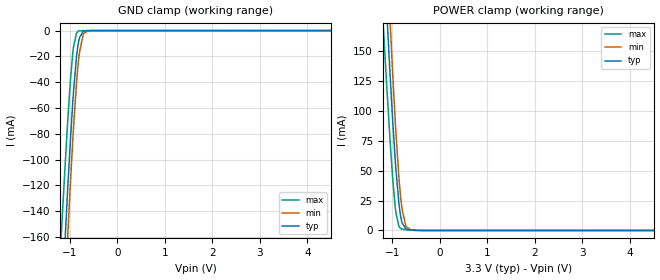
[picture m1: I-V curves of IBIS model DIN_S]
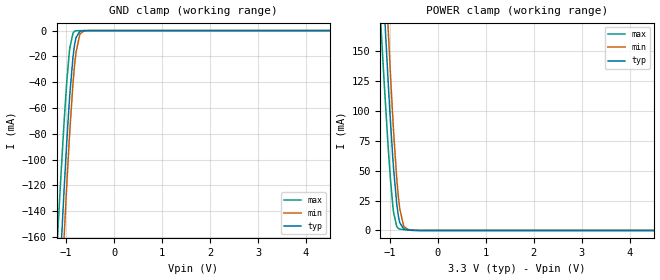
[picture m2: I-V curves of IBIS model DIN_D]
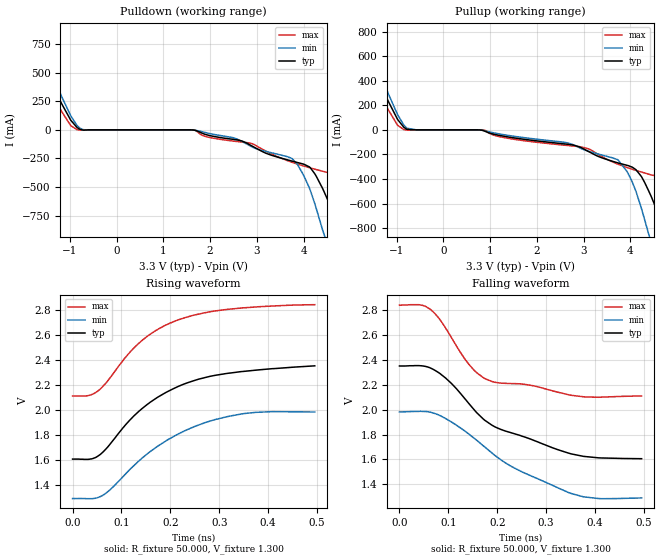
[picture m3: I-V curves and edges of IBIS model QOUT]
|Texas Instruments Incorporated
|3.3V  ECL 1:2 Fanout Buffer
|Valid for clock frequencies upto 2.4 - 2.9GHz
|*_S components are valid for parts used with D and DB in Single-Ended mode
|*_D components are valid for parts used with D and DB in Differential mode
| Marketing part#   Voltage Range   Package-type   #pins
|SN65LVEL11D   3.0V-3.8V   SOIC   8-pin
|SN65LVEL11DGK   3.0V-3.8V   MSOP(SOIC-TSSOP)   8-pin
[IBIS Ver]   4.0
[File name]   sn65lvel11.ibs
[File Rev]   1.1
[Date]   01/28/2009
[Source]   Texas Instruments Incorporated.
   Analog-eLab, HPA
   12500 TI Blvd
   Dallas, TX -75243
   For Support e-mail: elab_ibis@list.ti.com
[Notes]   Revision History:
   1.0: 01/27/2009
   - Model based on Simulations in TISPICE
   - Model not matched to silicon measurements
   1.1: 01/28/2009
   - Model updated with separate components and input_ECL models
   with *_S and *_D extensions. *_S valid for part configuration with
   D and DB as single-ended. *_D valid for part configuration with
   D and DB pair as differential
   - Updated ccomp, [pin] and [package] parasitics to be valid
   for speeds upto 2.9GHz
[Disclaimer]
 This product is designed as an aid for customers of Texas Instruments.
 No warranties, either expressed or implied, with respect to this third
 party software (if any) or with respect to its fitness for any
 particular purpose is claimed by Texas Instruments or the author. The
 software (if any) is provided solely on an "as is" basis. The entire
 risk as to its quality and performance is with the customer
[Copyright] (C) Copyright 2009 Texas Instruments Incorporated.
   All rights reserved.
|   SN65LVEL11D_S for D/DB configured as Single-ended
[Component]   SN65LVEL11D_S
[Manufacturer]  Texas Instruments Incorporated
[Package]   |8-pin SOIC
|   typ   min   max
R_pkg   0.317   0.222   0.412
L_pkg   2.169nH   1.866nH   2.472nH
C_pkg   0.429pF   0.393pF   0.466pF
[Pin]   signal_name   model_name   R_pin   L_pin   C_pin
1   Q0   QOUT   0.37987  2.46895nH   0.46661pF
2   Q0B   QOUT   0.41159  2.31383nH   0.39282pF
3   Q1   QOUT   0.41165  2.31858nH   0.39342pF
4   Q1B   QOUT   0.37973  2.47237nH   0.46538pF
5   VEE   GND   0.37987  2.47742nH   0.46746pF
6   DB   DIN_S   0.22226  1.88277nH   0.44363pF
7   D   DIN_S   0.22215  1.86618nH   0.44245pF
8   VCC   POWER   0.37988  2.46900nH   0.46723pF
|   SN65LVEL11DGK_S for D/DB configured as Single-ended
[Component]   SN65LVEL11DGK_S
[Manufacturer]  Texas Instruments Incorporated
[Package]   |8-pin SOIC-TSSOP(MSOP)
|   typ   min   max
R_pkg   0.254   0.173   0.335
L_pkg   1.629nH   1.447nH   1.811nH
C_pkg   0.413pF   0.388pF   0.438pF
[Pin]   signal_name   model_name   R_pin   L_pin   C_pin
1   Q0   QOUT   0.33466   1.80718nH   0.38798pF
2   Q0B   QOUT   0.31084   1.69655nH   0.40564pF
3   Q1   QOUT   0.31084   1.69710nH   0.40565pF
4   Q1B   QOUT   0.33466   1.81116nH   0.38809pF
5   VEE   GND   0.33466   1.81117nH   0.38874pF
6   DB   DIN_S   0.17319   1.44830nH   0.43798pF
7   D   DIN_S   0.17318   1.44692nH   0.43795pF
8   VCC   POWER   0.33466   1.80716nH   0.38864pF
[Diff_pin]   inv_pin   vdiff   tdelay_typ   tdelay_min   tdelay_max
| '1,3' pins are Diff_pin(s) and '2,4' pins respectively are inv_pin(s)
1   2   0.300   0   NA   NA
3   4   0.300   0   NA   NA
|   SN65LVEL11D_D for D/DB configured as Differential
[Component]   SN65LVEL11D_D
[Manufacturer]  Texas Instruments Incorporated
[Package]   |8-pin SOIC
|   typ   min   max
R_pkg   0.317   0.222   0.412
L_pkg   2.169nH   1.866nH   2.472nH
C_pkg   0.429pF   0.393pF   0.466pF
[Pin]   signal_name   model_name   R_pin   L_pin   C_pin
1   Q0   QOUT   0.37987  2.46895nH   0.46661pF
2   Q0B   QOUT   0.41159  2.31383nH   0.39282pF
3   Q1   QOUT   0.41165  2.31858nH   0.39342pF
4   Q1B   QOUT   0.37973  2.47237nH   0.46538pF
5   VEE   GND   0.37987  2.47742nH   0.46746pF
6   DB   DIN_D   0.22226  1.88277nH   0.44363pF
7   D   DIN_D   0.22215  1.86618nH   0.44245pF
8   VCC   POWER   0.37988  2.46900nH   0.46723pF
|   SN65LVEL11DGK_D for D/DB configured as Differential
[Component]   SN65LVEL11DGK_D
[Manufacturer]  Texas Instruments Incorporated
[Package]   |8-pin SOIC-TSSOP(MSOP)
|   typ   min   max
R_pkg   0.254   0.173   0.335
L_pkg   1.629nH   1.447nH   1.811nH
C_pkg   0.413pF   0.388pF   0.438pF
[Pin]   signal_name   model_name   R_pin   L_pin   C_pin
1   Q0   QOUT   0.33466   1.80718nH   0.38798pF
2   Q0B   QOUT   0.31084   1.69655nH   0.40564pF
3   Q1   QOUT   0.31084   1.69710nH   0.40565pF
4   Q1B   QOUT   0.33466   1.81116nH   0.38809pF
5   VEE   GND   0.33466   1.81117nH   0.38874pF
6   DB   DIN_D   0.17319   1.44830nH   0.43798pF
7   D   DIN_D   0.17318   1.44692nH   0.43795pF
8   VCC   POWER   0.33466   1.80716nH   0.38864pF
[Diff_pin]   inv_pin   vdiff   tdelay_typ   tdelay_min   tdelay_max
|  '1,3,7' pins are Diff_pin(s) and  '2,4,6' pins respectively are inv_pin(s)
1   2   0.300   0   NA   NA
3   4   0.300   0   NA   NA
7   6   0.750   0   NA   NA
| Models and submodels in the file (3): DIN_S (Input_ECL), DIN_D (Input_ECL), QOUT (Output_ECL)
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|   DIN_S Input_ECL MODEL for D/DB configured as Single-ended
[Model]   DIN_S
Model_type   Input_ECL
|Signals   D & DB pair  for 3.3V option
|Input Levels
Vinl = 1.6575V
Vinh = 2.2775V
|   typ   min   max
C_comp   0.4389pF   0.4995pF   0.3882pF
[Model Spec]
Vinl   1.6575V   1.490V   1.825V
Vinh   2.2775V   2.135V   2.420V
[Voltage Range]   3.3V   3.0V   3.8V
| Junction Temperature (Ambient temp is 25C typ, 85C min,  -40C max)
[Temperature Range]   40.0   100.0   -40.0
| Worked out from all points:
|   GND clamp passes 1 mA (typ) near -0.72 V on its own axis
|   POWER clamp passes 1 mA (typ) near -0.68 V on its own axis
[GND Clamp]
|   Voltage   I(typ)   I(min)   I(max)
-3.3V     -2.091A    -2.267A    -1.84A
-1.178V   -223.1mA   -268.1mA   -159.8mA
-1.114V   -174.9mA   -216.1mA   -116.4mA
-1.05V    -128.8mA   -166.2mA   -75.51mA
-1.031V   -115.6mA   -151.9mA   -64.11mA
-985.5mV  -85.75mA   -119.2mA   -39.37mA
-924.9mV  -50.43mA   -78.94mA   -14.21mA
-857.1mV  -20.62mA   -41.07mA   -2.058mA
-819.2mV  -9.937mA   -25.03mA   -387.8uA
-714.5mV  -575.7uA   -3.132mA   -15.22uA
-617.5mV  -32.2uA    -167uA     -11.93uA
6.6V      0A         0A         0A
[POWER Clamp]
|   Voltage   I(typ)   I(min)   I(max)
-3.3V     2.121A     2.694A     1.787A
-1.204V   254.8mA    320.6mA    183.7mA
-1.178V   233.9mA    296.2mA    165.4mA
-1.114V   183.2mA    237.2mA    120.8mA
-1.031V   120.9mA    165mA      67.08mA
-985.5mV  89.72mA    128.8mA    41.69mA
-924.9mV  52.95mA    84.5mA     15.92mA
-857.1mV  22.19mA    43.75mA    3.392mA
-819.2mV  11.22mA    26.76mA    1.543mA
-713.4mV  1.403mA    3.901mA    687.2uA
-501.9mV  169.5uA    262.7uA    25.44uA
6.6V      0A         0A         0A
|   DIN_D Input_ECL MODEL for D/DB configured as Differential
[Model]   DIN_D
Model_type   Input_ECL
|Signals   D & DB pair  for 3.3V option
|Input Levels
Vinl = 1.45V
Vinh = 2.20V
|   typ   min   max
C_comp   0.4389pF   0.4995pF   0.3882pF
[Model Spec]
Vinl   1.45V   0.65V   2.35V
Vinh   2.20V   1.40V   3.10V
[Voltage Range]   3.3V   3.0V   3.8V
| Junction Temperature (Ambient temp is 25C typ, 85C min,  -40C max)
[Temperature Range]   40.0   100.0   -40.0
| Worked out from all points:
|   GND clamp passes 1 mA (typ) near -0.72 V on its own axis
|   POWER clamp passes 1 mA (typ) near -0.68 V on its own axis
[GND Clamp]
|   Voltage   I(typ)   I(min)   I(max)
-3.3V     -2.091A    -2.267A    -1.84A
-1.178V   -223.1mA   -268.1mA   -159.8mA
-1.114V   -174.9mA   -216.1mA   -116.4mA
-1.05V    -128.8mA   -166.2mA   -75.51mA
-1.031V   -115.6mA   -151.9mA   -64.11mA
-985.5mV  -85.75mA   -119.2mA   -39.37mA
-924.9mV  -50.43mA   -78.94mA   -14.21mA
-857.1mV  -20.62mA   -41.07mA   -2.058mA
-819.2mV  -9.937mA   -25.03mA   -387.8uA
-714.5mV  -575.7uA   -3.132mA   -15.22uA
-617.5mV  -32.2uA    -167uA     -11.93uA
6.6V      0A         0A         0A
[POWER Clamp]
|   Voltage   I(typ)   I(min)   I(max)
-3.3V     2.121A     2.694A     1.787A
-1.204V   254.8mA    320.6mA    183.7mA
-1.178V   233.9mA    296.2mA    165.4mA
-1.114V   183.2mA    237.2mA    120.8mA
-1.031V   120.9mA    165mA      67.08mA
-985.5mV  89.72mA    128.8mA    41.69mA
-924.9mV  52.95mA    84.5mA     15.92mA
-857.1mV  22.19mA    43.75mA    3.392mA
-819.2mV  11.22mA    26.76mA    1.543mA
-713.4mV  1.403mA    3.901mA    687.2uA
-501.9mV  169.5uA    262.7uA    25.44uA
6.6V      0A         0A         0A
|   QOUT Output_ECL MODEL
[Model]   QOUT
Model_type   Output_ECL
| Signals   Q0/Q0B and Q1/Q1B pair  for 3.3V option
Cref = 0.0pF   |Timing specification test load capacitance value
Rref = 50.00Ohm
| variable   typ   min   max
C_comp   0.3584pF   0.4429pF   0.2713pF
[Model Spec]
Vref   1.3V   1.0V   1.8V
Vmeas   1.3V   1.0V   1.8V
[pullup reference]   3.3V   3.0V   3.8V
[pulldown reference]   3.3V   3.0V   3.8V
| Junction Temperature (Ambient temp is 25C typ, 85C min,  -40C max)
[Temperature Range]   40.0   100.0   -40.0
[Voltage Range]   3.3V   3.0V   3.8V
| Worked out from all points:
|   rising waveform, R_fixture 50.000, V_fixture 1.300: 20-80 % time 143ps typ, 142ps min, 124ps max; typ from 1.6 V to 2.35 V
|   falling waveform, R_fixture 50.000, V_fixture 1.300: 20-80 % time 165ps typ, 164ps min, 83.9ps max; typ from 2.35 V to 1.6 V
[Pulldown]
|   Voltage   I(typ)   I(min)   I(max)
-3.3V     2.102A     2.676A     1.767A
-2.168V   1.086A     1.352A     900.5mA
-1.97V    910.8mA    1.128A     750.3mA
-1.772V   736.4mA    907.8mA    600.7mA
-843.8mV  19.66mA    37.12mA    1.247mA
1.651V    -1.982mA   -2.161mA   -1.339mA
2.879V    -136.9mA   -145.2mA   -117.6mA
3.865V    -284.9mA   -298.8mA   -298.4mA
4.417V    -519.1mA   -885mA     -362.4mA
4.791V    -915.1mA   -1.31A     -441.1mA
5.32V     -1.453A    -1.899A    -854.4mA
6.6V      -2.863A    -3.466A    -2.014A
[Pullup]
|   Voltage   I(typ)   I(min)   I(max)
-3.3V     2.102A     2.676A     1.767A
-2.168V   1.086A     1.352A     900.5mA
-1.772V   736.4mA    907.8mA    600.7mA
-843.8mV  19.66mA    37.12mA    1.247mA
849.8mV   -5.841mA   -5.085mA   -599.9uA
3.051V    -166.1mA   -167.9mA   -148.5mA
3.728V    -268.8mA   -243.1mA   -278.9mA
3.925V    -288.6mA   -337.6mA   -306.5mA
4.378V    -486.3mA   -830.6mA   -359.6mA
4.736V    -857.4mA   -1.247A    -413.3mA
5.302V    -1.435A    -1.879A    -839.8mA
6.6V      -2.936A    -3.754A    -2.034A
[Ramp]
R_load = 50.00Ohm
|   typ   min   max
dV/dt_r   422.100mV/142.967ps 345.681mV/142.245ps 433.060mV/124.230ps
dV/dt_f   435.179mV/165.646ps 335.670mV/163.829ps 431.437mV/84.694ps
[Rising Waveform]
R_fixture = 50.000
V_fixture = 1.300
V_fixture_min = 1.000
V_fixture_max = 1.800
|  time   V(typ)   V(min)   V(max)
0s        1.605V     1.289V     2.111V
34.55ps   1.604V     1.288V     2.116V
61.5ps    1.659V     1.314V     2.185V
105.9ps   1.868V     1.476V     2.409V
134.6ps   1.984V     1.587V     2.53V
171.2ps   2.093V     1.7V       2.637V
216.6ps   2.188V     1.807V     2.721V
270.8ps   2.258V     1.897V     2.777V
346.1ps   2.306V     1.967V     2.816V
495.5ps   2.352V     1.982V     2.842V
[Falling Waveform]
R_fixture = 50.000
V_fixture = 1.300
V_fixture_min = 1.000
V_fixture_max = 1.800
|  time   V(typ)   V(min)   V(max)
0s        2.352V     1.982V     2.842V
42.78ps   2.354V     1.987V     2.844V
64.86ps   2.333V     1.978V     2.803V
95.66ps   2.251V     1.926V     2.65V
141.9ps   2.05V      1.804V     2.366V
189.2ps   1.875V     1.651V     2.227V
237.1ps   1.804V     1.526V     2.21V
351.3ps   1.644V     1.325V     2.116V
407.7ps   1.612V     1.284V     2.1V
495.5ps   1.605V     1.289V     2.111V
